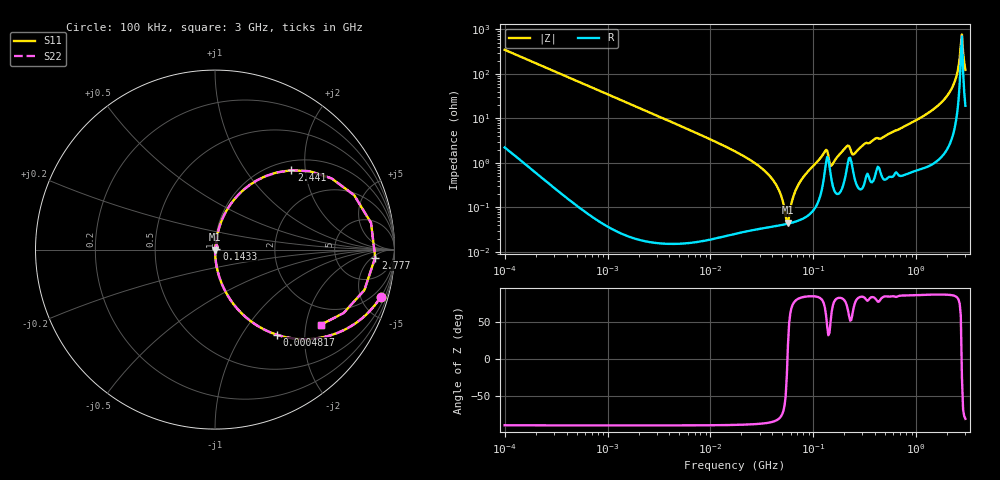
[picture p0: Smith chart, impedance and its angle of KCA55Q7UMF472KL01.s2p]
!Murata Part Number: KCA55Q7UMF472KL01
!These Parameters are Measured in Series Mode Connection
!Data Generated on Jan 08, 2026
!  o--ll--o
!Port1  Port2
!  o------o
!Operation Temp=25[degC], DC Bias Voltage=0[V]
!Freq. Start=100[kHz] Stop=3[GHz] 401[Steps]
# Hz S RI R 50
!Freq.(Hz) S11(Real) S11(Imag) S21(Real) S21(Imag) S12(Real) S12(Imag) S22(Real) S22(Imag)
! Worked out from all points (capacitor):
!   401 points, 100 kHz to 3 GHz, reference 50 ohm
!   read as one part in series: C = 4.56 nF near 105.3 kHz
!   lowest |Z| = 45.7 mohm at 56.68 MHz (marker M1)
!   series resonance near 56 MHz, so ESL is about 1.8 nH
!   S11 on the Smith chart (normalised r, x): 100 kHz: 1.04, -6.97; 481.7 kHz: 1.00, -1.45; 143.3 MHz: 1.02, +0.01; 2.441 GHz: 1.19, +1.69; 2.777 GHz: 15, -7; 3 GHz: 1.38, -2.43
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100000  0.9226 -0.2641  0.0774 0.2641  0.0774 0.2641  0.9226 -0.2641
481683  0.3448 -0.4745  0.6552 0.4745  0.6552 0.4745  0.3448 -0.4745
562235  0.2787 -0.4476  0.7213 0.4476  0.7213 0.4476  0.2787 -0.4476
3161081  0.0121 -0.1088  0.9879 0.1088  0.9879 0.1088  0.0121 -0.1088
1.77727e7  0.000567 -0.0176  0.9994 0.0176  0.9994 0.0176  0.000567 -0.0176
3.951212e7  0.000386 -0.00445  0.9996 0.00445  0.9996 0.00445  0.000386 -0.00445
4.611977e7  0.000396 -0.00245  0.9996 0.00245  0.9996 0.00245  0.000396 -0.00245
5.667996e7  0.00043 0.000153  0.9996 -0.000153  0.9996 -0.000153  0.00043 0.000153
6.965816e7  0.000501 0.00284  0.9995 -0.00284  0.9995 -0.00284  0.000501 0.00284
9.738194e7  0.000861 0.00805  0.9991 -0.00805  0.9991 -0.00805  0.000861 0.00805
1.293002e8  0.00669 0.0168  0.9933 -0.0168  0.9933 -0.0168  0.00669 0.0168
1.43341e8  0.00834 0.00576  0.9917 -0.00576  0.9917 -0.00576  0.00834 0.00576
1.548634e8  0.00304 0.00919  0.997 -0.00919  0.997 -0.00919  0.00304 0.00919
2.109903e8  0.00763 0.0221  0.9924 -0.0221  0.9924 -0.0221  0.00763 0.0221
2.52704e8  0.00457 0.0157  0.9954 -0.0157  0.9954 -0.0157  0.00457 0.0157
5.475153e8  0.00687 0.0448  0.9931 -0.0448  0.9931 -0.0448  0.00687 0.0448
1.7917e9  0.0665 0.2212  0.9335 -0.2212  0.9335 -0.2212  0.0665 0.2212
2.145926e9  0.1643 0.3375  0.8357 -0.3375  0.8357 -0.3375  0.1643 0.3375
2.441062e9  0.4262 0.4424  0.5738 -0.4424  0.5738 -0.4424  0.4262 0.4424
2.570185e9  0.6504 0.3964  0.3496 -0.3964  0.3496 -0.3964  0.6504 0.3964
2.776789e9  0.8926 -0.0441  0.1074 0.0441  0.1074 0.0441  0.8926 -0.0441
3e9  0.5883 -0.4193  0.4117 0.4193  0.4117 0.4193  0.5883 -0.4193
